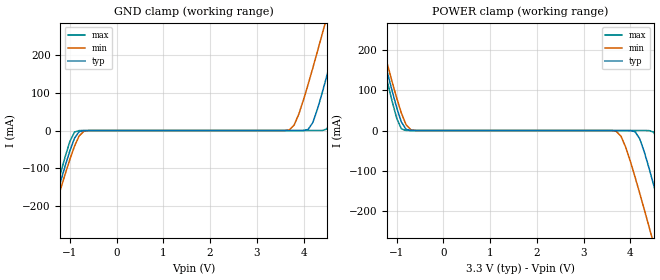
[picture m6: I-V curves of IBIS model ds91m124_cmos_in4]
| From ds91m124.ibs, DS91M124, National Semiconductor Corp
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|   Model  ds91m124_cmos_in4
[Model]   ds91m124_cmos_in4
Model_type Input
Vinh=2.0
Vinl=0.8
|   Typ   Min   Max
C_comp   2.132p   2.099p   2.164p
[Model Spec]
S_overshoot_high   3.3   3.0   3.6
S_overshoot_low   0.0   0.0   0.0
[Temperature Range]   25   85   -40
[Voltage Range]   3.3   3.0   3.6
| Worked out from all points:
|   GND clamp passes 1 mA (typ) near -0.73 V on its own axis
|   POWER clamp passes 1 mA (typ) near -0.73 V on its own axis
[GND Clamp]
-3.3V     -1.101A    -1.073A    -1.137A
-1.5V     -269.1mA   -282.5mA   -255mA
-1V       -54.13mA   -76.92mA   -29.38mA
-800mV    -2.939mA   -14.27mA   -73.89uA
3.7V      2.201nA    2.178mA    6.448pA
3.9V      3.125uA    43.51mA    7.288pA
4.1V      2.971mA    122.6mA    74.72pA
4.4V      99.8mA     255.1mA    73.92uA
4.5V      145.1mA    300.5mA    4.124mA
4.8V      287.3mA    438.7mA    121.9mA
5.1V      433.3mA    578.6mA    273.4mA
6.5V      1.128A     1.24A      1.009A
[POWER Clamp]
-3.3V     1.178A     1.145A     1.062A
-1.5V     287.3mA    300.5mA    273.4mA
-1.4V     239.3mA    255.1mA    222.1mA
-1V       57.18mA    81.21mA    30.95mA
-800mV    2.971mA    14.69mA    73.92uA
3.7V      -2.203nA   -2.162mA   -7.62pA
4.1V      -2.939mA   -115.7mA   -75.9pA
4.4V      -93.98mA   -239.9mA   -73.89uA
4.5V      -136.3mA   -282.5mA   -4.054mA
4.8V      -269.1mA   -411.9mA   -114mA
5.1V      -405.5mA   -542.9mA   -255mA
6.5V      -1.054A    -1.073A    -939.2mA
